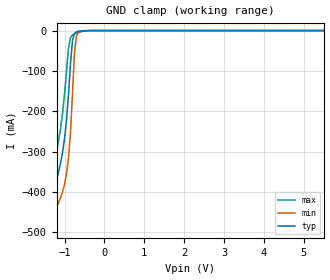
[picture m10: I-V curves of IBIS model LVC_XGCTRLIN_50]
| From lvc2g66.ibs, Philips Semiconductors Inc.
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|   Model LVC_XGCTRLIN_50
[Model]   LVC_XGCTRLIN_50
Model_type   Input
Vinl =   1.5V
Vinh =   3.5V
C_comp   2.89pF   1.97pF   3.94pF
[Model Spec]
| Note: The input and output voltage ratings may be exceeded if the input and
|   output current ratings are observed (please refer to the data sheet)
|   Subparameter   typ   min   max
| Thresholds
Vinh   3.5   3.15   3.85
Vinl   1.5   1.35   1.65
| Overshoot
S_overshoot_high   6.5   6.5   6.5   | Static overshoot
S_overshoot_low   -0.5   -0.5   -0.5
D_overshoot_high   11.0   11.0   11.0   | Dynamic overshoot
D_overshoot_low   -0.95   -0.9   -1.0
D_overshoot_time   3n   3n   3n
|Ambient temperature:   25   85   -40
[Temperature Range]   50   105   -10
[Voltage Range]   5.0V   4.5V   5.5V
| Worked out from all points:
|   GND clamp passes 1 mA (typ) near -0.59 V on its own axis
|Process Range   nominal   slow   fast
[GND_clamp]
| voltage   I(typ)   I(min)   I(max)
-5.5V     -4.585A    -4.637A    -4.534A
-1.45V    -567.8mA   -628.4mA   -505.9mA
-1.4V     -520.6mA   -581.5mA   -458.5mA
-1.3V     -430.1mA   -491.9mA   -367mA
-1.2V     -369.6mA   -437.9mA   -299.9mA
-1.05V    -303mA     -399.7mA   -205.6mA
-950mV    -222.3mA   -354.8mA   -100.4mA
-850mV    -82.04mA   -253.9mA   -17.37mA
-800mV    -24.94mA   -156mA     -10.72mA
-750mV    -6.792mA   -54.58mA   -8.095mA
-700mV    -2.837mA   -13.44mA   -6.14mA
5.5V      1.794nA    5.479nA    963.8pA
